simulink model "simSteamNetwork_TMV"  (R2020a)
settings: Solver=ode15s  StartTime=0.0  StopTime=tsim  RelTol=1e-8
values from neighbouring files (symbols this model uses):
  dp0 = 2    [Main.m]
  dpH = 1    [Main.m]
  dpHC = 1    [Main.m]
  dpL = -0.5    [Main.m]
  dpLC1 = -0.5    [Main.m]
  dpLC2 = -0.5    [Main.m]
  dTH = 0    [Main.m]
  dvH = 0;-AH*dpH    [Main.m]
  dvL = 0;-AL*dpL    [Main.m]
  dzHC = 0    [Main.m]
  dzLC1 = 0    [Main.m]
  dzLC2 = 0    [Main.m]
  KcH = 1/(tauCH+thetaH)    [Main.m]
  KcL = 1/(tauCL+thetaL)    [Main.m]
  nd = size(d0,2)    [Main.m]    (also in Main_OL.m; runTestCalcBlk.m; runTransf.m; runTransfOL.m)
  np = size(p,2)    [Main.m]    (also in runH2Psim.m = length(param); Main_OL.m; runTestCalcBlk.m; runTransf.m)
  nu = 1    [Main.m]    (also in runH2Psim.m = length(u0); Main_OL.m; runTestCalcBlk.m; runTransf.m)
  nx = size(x0,1)    [Main.m]    (also in H2P_Turbine_driven.m = param(end); runTD.m = length(x0); H2P_Boiler_driven.m = param(end); runBD.m = length(x0))
  p0 = d(4)    [CalcBlk.m]    (also in SteadyStateCond.m = 42; SteamNetwork.m)
  param = [R;gamma;VH;VL;phi;CvH;CvHC;CvTB;CvLC1;CvLC2;AH;AL]    [Main.m]    (also in runTD.m = [Tref;TrefB;dHvap;cpg;cpW;cpSt;R;Mwt;     T0;TG0;ME;pC;     ; runBD.m = [Tref;TrefB;dHvap;cpg;cpW;cpSt;R;Mwt;          T0;TG0;ME;pC;; runFP.m = [Tref;TrefB;dHvap;cpg;cpW;cpSt;R;Mwt;          T0;TG0;ME;pC;; runFPV2.m = [Tref;TrefB;dHvap;cpg;cpW;cpSt;R;Mwt;          T0;TG0;ME;pC;)
  pH0 = 40    [SteadyStateCond.m]
  pHC0 = 38    [SteadyStateCond.m]
  pL0 = 7    [SteadyStateCond.m]
  pLC10 = 6    [SteadyStateCond.m]
  pLC20 = 5    [SteadyStateCond.m]
  tauIH = min(tauH,4*(tauCH+thetaH))    [Main.m]
  tauIL = min(tauL,4*(tauCL+thetaL))    [Main.m]
  TH0 = 380+273    (= 653)    [SteadyStateCond.m]
  tp0 = 10    [Main.m]
  tpHC = 20    [Main.m]
  tpLC1 = 30    [Main.m]
  tpLC2 = 40    [Main.m]
  tspH = 50    [Main.m]
  tspL = 60    [Main.m]
  tTH = 0    [Main.m]
  tzHC = 0    [Main.m]
  tzLC1 = 0    [Main.m]
  tzLC2 = 0    [Main.m]
  v0H = -AH*pH0    [Main.m]
  v0L = -AL*pL0    [Main.m]
  x0 = [Tcend(1:N)'; Thend(1:N)']    [Main.m]    (also in runTD.m = [TE0;TD0;TSh0;MD0; MSh0;w0;TA0;0;0;0;0;0;0;0;0;0]; runBD.m = [TE0;TD0;TSh0;MD0; MSh0;w0;TA0;0;0;0;0;0;0;0;0;0]; runFP.m = [TE0;TD0;TSh0;MD0; MSh0;w0;TA0;0;0;0;0;0;0;0]; runFPV2.m = [TE0;TD0;TSh0;MD0; MSh0;w0;TA0;0;0;0;0;0;0;0])
  z0 = 0.5    [SteadyStateCond.m]    (also in runTD.m = [TGE0;TGD;TGSh;pT; Pm0;mG;zV]; runBD.m = [TGE0;TGD;TGSh;pT; Pm0;mG;zV]; runFP.m = [TGE0;TGD;TGSh;pT; Pm0;mG;zV]; runFPV2.m = [TGE0;TGD;TGSh;pT; Pm0;mG;zV])
undefined symbols (not defined in the file or in its folder): CalcBlk, SteamNetwork

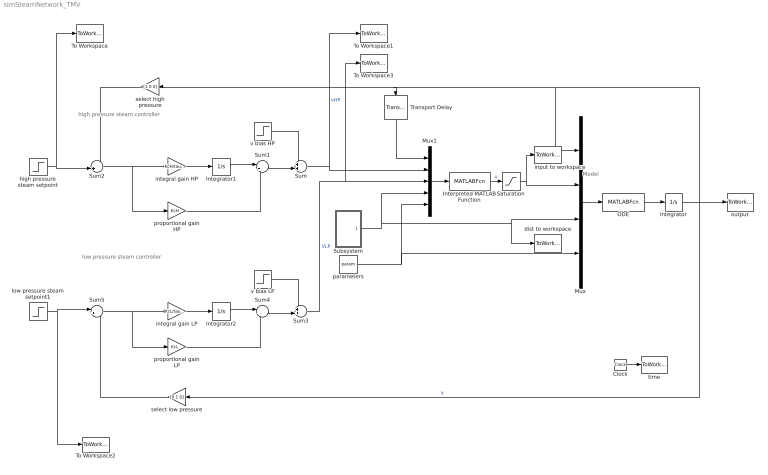
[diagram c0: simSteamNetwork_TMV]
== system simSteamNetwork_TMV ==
  note: Model
  note: low pressure steam controller
  note: high pressure steam controller
  Clock : Clock
  Integrator : Integrator  InitialCondition=x0
  Integrator1 : Integrator
  Integrator2 : Integrator
  Interpreted MATLAB Function : MATLABFcn  MATLABFcn=CalcBlk(u(1:nx),(u(nx+1:nx+nu)),u(nx+nu+1:nx+nu+nd),u(nx+nu+nd+1:nx+nu+nd+np))
  Mux : Mux
  Mux1 : Mux  Inputs=5
  ODE : MATLABFcn  MATLABFcn=SteamNetwork(u(1:nx),(u(nx+1:nx+nu)),u(nx+nu+1:nx+nu+nd),u(nx+nu+nd+1:nx+nu+nd+np))
  Saturation : Saturate  UpperLimit=1  LowerLimit=0
  Subsystem : Subsystem
  Sum : Sum  Inputs=++|
  Sum1 : Sum  Inputs=|++
  Sum2 : Sum  Inputs=-+|
  Sum3 : Sum  Inputs=++|
  Sum4 : Sum  Inputs=|++
  Sum5 : Sum  Inputs=|+-
  To Workspace : ToWorkspace  VariableName=pHsp  SampleTime=-1
  To Workspace1 : ToWorkspace  VariableName=vH  SampleTime=-1
  To Workspace2 : ToWorkspace  VariableName=pLsp  SampleTime=-1
  To Workspace3 : ToWorkspace  VariableName=vL  SampleTime=-1
  Transport Delay : TransportDelay  InitialOutput=x0
  dist to workspace : ToWorkspace  VariableName=d  SampleTime=-1
  high pressure steam setpoint : Step  Time=tspH  Before=pH0  After=pH0+dpH  SampleTime=0
  input to workspace : ToWorkspace  VariableName=u  SampleTime=-1
  integral gain HP : Gain  Gain=KcH/tauIH  Multiplication=Matrix(K*u)
  integral gain LP : Gain  Gain=KcL/tauIL  Multiplication=Matrix(K*u)
  low pressure steam setpoint1 : Step  Time=tspL  Before=pL0  After=pL0+dpL  SampleTime=0
  output : ToWorkspace  VariableName=y  SampleTime=-1
  parameters : Constant  Value=param
  proportional gain HP : Gain  Gain=KcH  Multiplication=Matrix(K*u)
  proportional gain LP : Gain  Gain=KcL  Multiplication=Matrix(K*u)
  select high pressure : Gain  Gain=[1 0 0]  Multiplication=Matrix(K*u)
  select low pressure : Gain  Gain=[0 1 0]  Multiplication=Matrix(K*u)
  time : ToWorkspace  VariableName=time  SampleTime=-1
  v bias HP : Step  Time=tspH  Before=v0H  After=v0H+dvH  SampleTime=0
  v bias LP : Step  Time=tspL  Before=v0L  After=v0L+dvL  SampleTime=0
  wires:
  ODE/1 -> Integrator/1
  Integrator/1 -> Mux/1, Transport Delay/1, select high pressure/1, select low pressure/1, output/1  "y"
  Mux/1 -> ODE/1
  Interpreted MATLAB Function/1 -> Saturation/1  "u"
  parameters/1 -> Mux/4, Mux1/5
  Clock/1 -> time/1
  Sum/1 -> To Workspace1/1, Mux1/2  "vHP"
  v bias HP/1 -> Sum/1
  Integrator1/1 -> Sum1/1
  integral gain HP/1 -> Integrator1/1
  Sum1/1 -> Sum/2
  proportional gain HP/1 -> Sum1/2
  Sum2/1 -> proportional gain HP/1, integral gain HP/1
  Mux1/1 -> Interpreted MATLAB Function/1
  Sum3/1 -> To Workspace3/1, Mux1/3  "VLP"
  integral gain LP/1 -> Integrator2/1
  Sum5/1 -> proportional gain LP/1, integral gain LP/1
  Integrator2/1 -> Sum4/1
  v bias LP/1 -> Sum3/1
  proportional gain LP/1 -> Sum4/2
  Sum4/1 -> Sum3/2
  high pressure steam setpoint/1 -> To Workspace/1, Sum2/2
  low pressure steam setpoint1/1 -> To Workspace2/1, Sum5/1
  select high pressure/1 -> Sum2/1
  select low pressure/1 -> Sum5/2
  Saturation/1 -> Mux/2, input to workspace/1
  Subsystem/1(u) -> Mux1/4, dist to workspace/1, Mux/3
  Transport Delay/1 -> Mux1/1

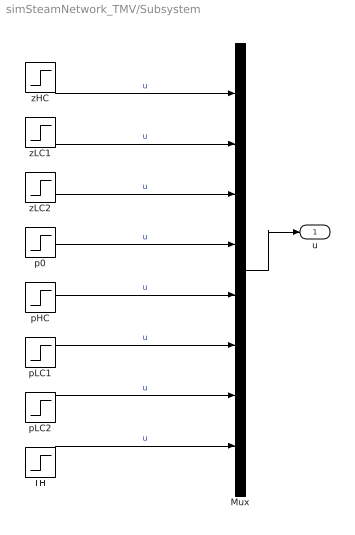
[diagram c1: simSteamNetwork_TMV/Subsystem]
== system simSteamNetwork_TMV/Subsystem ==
  Mux : Mux  Inputs=8
  TH : Step  Time=tTH  Before=TH0  After=TH0+dTH  SampleTime=0
  p0 : Step  Time=tp0  Before=p0  After=p0+dp0  SampleTime=0
  pHC : Step  Time=tpHC  Before=pHC0  After=pHC0+dpHC  SampleTime=0
  pLC1 : Step  Time=tpLC1  Before=pLC10  After=pLC10+dpLC1  SampleTime=0
  pLC2 : Step  Time=tpLC2  Before=pLC20  After=pLC20+dpLC2  SampleTime=0
  zHC : Step  Time=tzHC  Before=z0  After=z0+dzHC  SampleTime=0
  zLC1 : Step  Time=tzLC1  Before=z0  After=z0+dzLC1  SampleTime=0
  zLC2 : Step  Time=tzLC2  Before=z0  After=z0+dzLC2  SampleTime=0
  u : Outport
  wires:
  Mux/1 -> u/1
  zHC/1 -> Mux/1  "u"
  zLC1/1 -> Mux/2  "u"
  zLC2/1 -> Mux/3  "u"
  p0/1 -> Mux/4  "u"
  pHC/1 -> Mux/5  "u"
  pLC1/1 -> Mux/6  "u"
  pLC2/1 -> Mux/7  "u"
  TH/1 -> Mux/8  "u"
